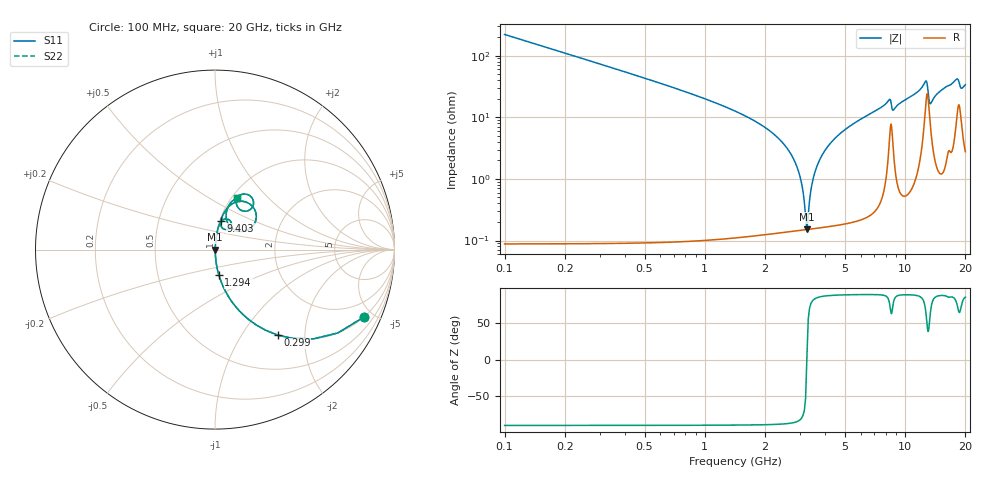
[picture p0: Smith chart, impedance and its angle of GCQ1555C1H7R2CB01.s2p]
!Murata Part Number: GCQ1555C1H7R2CB01
!These Parameters are Measured in Series Mode Connection
!Data Generated on Jan 08, 2026
!  o--ll--o
!Port1  Port2
!  o------o
!Operation Temp=25[degC], DC Bias Voltage=0[V]
!Freq. Start=100[MHz] Stop=20[GHz] 401[Steps]
# Hz S RI R 50
!Freq.(Hz) S11(Real) S11(Imag) S21(Real) S21(Imag) S12(Real) S12(Imag) S22(Real) S22(Imag)
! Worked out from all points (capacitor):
!   401 points, 100 MHz to 20 GHz, reference 50 ohm
!   read as one part in series: C = 7.2 pF near 199.5 MHz
!   lowest |Z| = 151 mohm at 3.234 GHz (marker M1)
!   series resonance near 3.231 GHz, so ESL is about 340 pH
!   S11 on the Smith chart (normalised r, x): 100 MHz: 1.00, -4.42; 299 MHz: 1.00, -1.47; 1.294 GHz: 1.00, -0.29; 9.403 GHz: 1.01, +0.34; 20 GHz: 1.06, +0.67
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1e8  0.8297 -0.3757  0.1703 0.3757  0.1703 0.3757  0.8297 -0.3757
2.99e8  0.3496 -0.4763  0.6504 0.4763  0.6504 0.4763  0.3496 -0.4763
5.975e8  0.1138 -0.3163  0.8862 0.3163  0.8862 0.3163  0.1138 -0.3163
1.294e9  0.0212 -0.1402  0.9788 0.1402  0.9788 0.1402  0.0212 -0.1402
2.687e9  0.00204 -0.0253  0.998 0.0253  0.998 0.0253  0.00204 -0.0253
2.93575e9  0.00162 -0.0131  0.9984 0.0131  0.9984 0.0131  0.00162 -0.0131
3.13475e9  0.0015 -0.00416  0.9985 0.00416  0.9985 0.00416  0.0015 -0.00416
3.23425e9  0.0015 0.000122  0.9985 -0.000122  0.9985 -0.000122  0.0015 0.000122
3.43325e9  0.00161 0.00831  0.9984 -0.00831  0.9984 -0.00831  0.00161 0.00831
3.7815e9  0.00208 0.0217  0.9979 -0.0217  0.9979 -0.0217  0.00208 0.0217
4.3785e9  0.00353 0.0424  0.9965 -0.0424  0.9965 -0.0424  0.00353 0.0424
6.7665e9  0.0158 0.1141  0.9842 -0.1141  0.9842 -0.1141  0.0158 0.1141
8.30875e9  0.0633 0.1708  0.9367 -0.1708  0.9367 -0.1708  0.0633 0.1708
8.70675e9  0.0465 0.1158  0.9535 -0.1158  0.9535 -0.1158  0.0465 0.1158
9.40325e9  0.0331 0.1617  0.9669 -0.1617  0.9669 -0.1617  0.0331 0.1617
1.005e10  0.0408 0.1845  0.9593 -0.1845  0.9593 -0.1845  0.0408 0.1845
1.2637e10  0.1998 0.2497  0.8002 -0.2497  0.8002 -0.2497  0.1998 0.2497
1.338325e10  0.0843 0.1283  0.9157 -0.1283  0.9157 -0.1283  0.0843 0.1283
1.67165e10  0.1182 0.2832  0.8818 -0.2832  0.8818 -0.2832  0.1182 0.2832
1.8408e10  0.2148 0.2585  0.7852 -0.2585  0.7852 -0.2585  0.2148 0.2585
1.9005e10  0.1444 0.2199  0.8556 -0.2199  0.8556 -0.2199  0.1444 0.2199
2e10  0.1212 0.2879  0.8788 -0.2879  0.8788 -0.2879  0.1212 0.2879
